{attribute 'no_assign'}
FUNCTION_BLOCK FB_DO_IED_MUnn_UnnATVTR1_VolSv EXTENDS FB_AcsiCommonDataClass
VAR_INPUT
	instMag: FB_AcsiDATypeAnalogueValue := (Fc:=ACSI_FC_MX, f:=(bPresence:=FALSE), bLinkResult:=THIS^.AddDataToContainer(ipData:=instMag));
	q: FB_AcsiDATypeQuality := (Fc:=ACSI_FC_MX, TrgOp:=ACSI_TrgOp_qchg, bLinkResult:=THIS^.AddDataToContainer(ipData:=q));
	units: FB_AcsiDATypeUnit := (Fc:=ACSI_FC_CF, TrgOp:=ACSI_TrgOp_dchg, SIUnit:=(eValue:=E_AcsiSIUnit.Volt), multiplier:=(eValue:=E_AcsiMultiplier.Hecto, bPresence:=TRUE), bLinkResult:=THIS^.AddDataToContainer(ipData:=units));
	sVC: FB_AcsiDATypeScaledValueConfig := (Fc:=ACSI_FC_CF, TrgOp:=ACSI_TrgOp_dchg, scaleFactor:=(fValue:=0.01), bLinkResult:=THIS^.AddDataToContainer(ipData:=sVC));
END_VAR
VAR
END_VAR

END_FUNCTION_BLOCK
